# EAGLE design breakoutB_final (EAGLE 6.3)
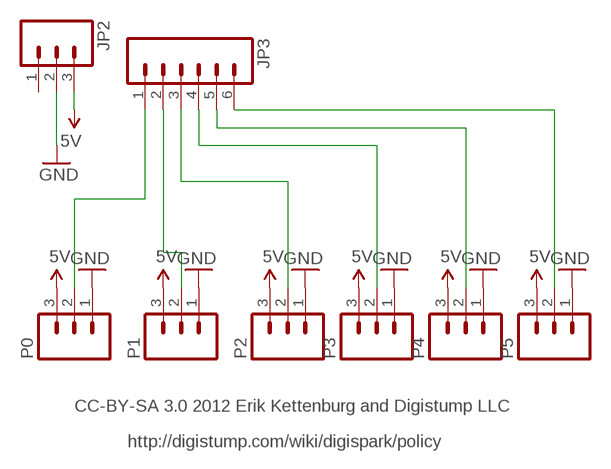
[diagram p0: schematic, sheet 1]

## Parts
JP2  M03PTH  [1X03]
JP3  M06SIP  [1X06]
P0  M03PTH  [1X03]
P1  M03PTH  [1X03]
P2  M03PTH  [1X03]
P3  M03PTH  [1X03]
P4  M03PTH  [1X03]
P5  M03PTH  [1X03]

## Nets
5V: JP2.3 P0.3 P1.3 P2.3 P3.3 P4.3 P5.3
GND: JP2.2 P0.1 P1.1 P2.1 P3.1 P4.1 P5.1
N$1: JP3.1 P0.2
N$2: JP3.2 P1.2
N$3: JP3.3 P2.2
N$4: JP3.4 P3.2
N$5: JP3.5 P4.2
N$6: JP3.6 P5.2
Unconnected: JP2.1

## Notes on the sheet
- CC-BY-SA 3.0 2012 Erik Kettenburg and Digistump LLC
- http://digistump.com/wiki/digispark/policy

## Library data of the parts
JP2 P0 P1-P5 = SparkFun:M03: Header 3 Standard 3-pin 0.1" header. Use with straight break away headers (SKU : PRT-00116), right angle break away headers (PRT-00553), swiss pins (PRT-00743), machine pins (PRT-00117), and female headers (PRT-00115). Molex polarized connector foot print use with SKU : PRT-08232 with associated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
JP3 = SparkFun:M06: Header 6 Standard 6-pin 0.1" header. Use with straight break away headers (SKU : PRT-00116), right angle break away headers (PRT-00553), swiss pins (PRT-00743), machine pins (PRT-00117), and female headers (PRT-00115). Molex polarized connector foot print use with SKU : PRT-08094 with associated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

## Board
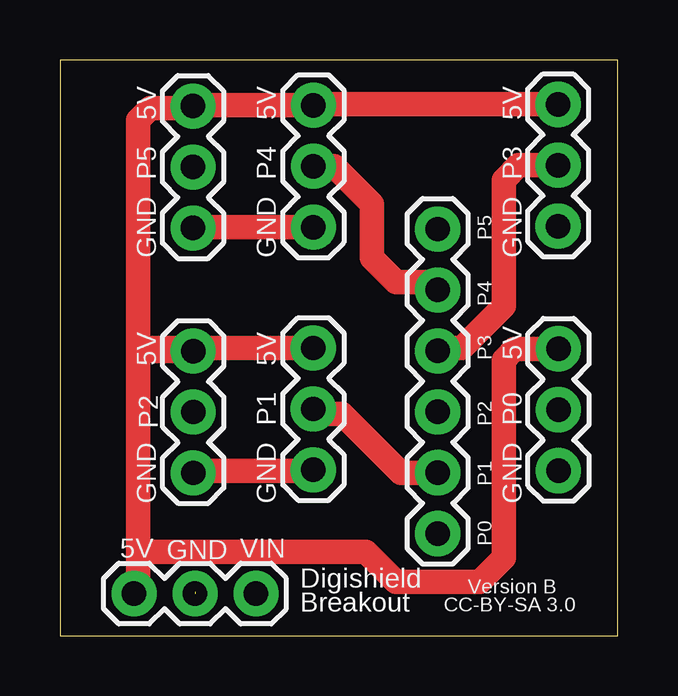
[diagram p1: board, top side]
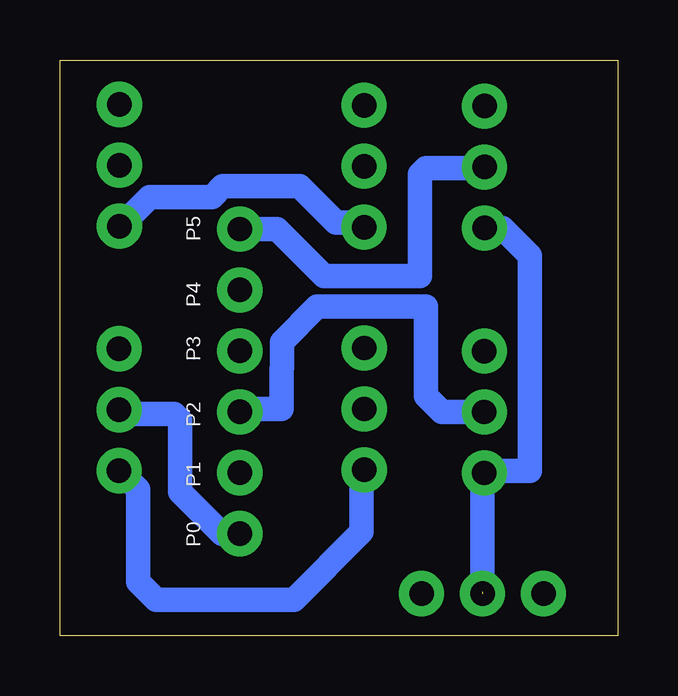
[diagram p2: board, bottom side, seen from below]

Size 23.25 x 24 mm. Coordinates in mm from the lower left corner, seen from the top.
Outline: 0,24 0,0 23.25,0 23.25,24 0,24
Copper layers (1*16): Top 0.0356mm / dielectric 1.5011mm / Bottom 0.0356mm
Design rules "default": minimum track width 40mil, minimum drill 40mil, track to track 8mil, track to pad 8mil, pad to pad 8mil, via to via 8mil, smd to smd 8mil, copper to edge 15mil, drill to drill 12mil, minimum pad ring 7mil, minimum via ring 7mil, stop-mask expansion 4mil, vias tented up to drill 25mil, thermal gap 10mil

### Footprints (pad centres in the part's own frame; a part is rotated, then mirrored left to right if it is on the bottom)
1X03 = drill 1.016 pad 1.88: 1 0,0; 2 2.54,0; 3 5.08,0
1X06 = drill 1.016 pad 1.88: 1 0,0; 2 2.54,0; 3 5.08,0; 4 7.62,0; 5 10.16,0; 6 12.7,0

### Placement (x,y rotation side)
JP2  8.17,1.75 180 top
JP3  15.75,4.25 90 top
P0  20.79,6.88 90 top
P1  10.56,6.91 90 top
P2  5.56,6.78 90 top
P3  20.77,17.07 90 top
P4  10.57,17.03 90 top
P5  5.55,17 90 top

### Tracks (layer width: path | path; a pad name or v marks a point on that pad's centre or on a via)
5V
  Top 1.016: P3.3 10.57,22.15 P4.3 5.55,22.11 P5.3 5.47,22 3.75,22 3.25,21.5 3.25,11.75 | 3.36,11.86 P2.3 5.56,11.99 P1.3 3.49,11.99 3.36,11.86 | 3.36,11.86 3.25,11.75 | 3.25,11.75 3.25,3.25 | 3.25,3.25 3.25,1.91 JP2.3 | P0.3 18.96,11.96 18.5,11.5 18.5,3.25 17.5,2.25 14,2.25 12.75,3.5 3.5,3.5 3.25,3.25
GND  (1 unrouted)
  Top 1.016: P1.1 10.52,6.86 5.64,6.86 P2.1 5.64,6.4 | P4.1 5.58,17.03 P5.1
  Bottom 1.016: 5.64,17.07 P5.1 4.8,17 3.66,15.85 3.66,6.86 5.49,6.86 P2.1 5.64,6.7 5.64,1.83 | 10.52,17.07 P4.1 10.97,17.22 11.73,17.22 13.26,18.75 16.46,18.75 16.92,18.29 19.51,18.29 20.73,17.07 P3.1 | P0.1 20,6.09 20,2.25 19.25,1.5 13.5,1.5 10.67,4.33 10.67,6.8 P1.1
N$1
  Bottom 1.016: JP3.1 16.5,4.25 18.25,6 18.25,9 18.5,9.25 20.62,9.25 P0.2
N$2
  Top 1.016: JP3.2 14.21,6.79 11.75,9.25 10.76,9.25 P1.2
N$3
  Bottom 1.016: JP3.3 15.7,9.45 14.02,9.45 14.02,11.12 14,11.15 14,12.25 12.53,13.72 8,13.72 8,10 7.32,9.32 P2.2
N$4
  Top 1.016: P3.2 19.11,19.61 18.5,19 18.5,13.75 16.75,12 15.88,12 JP3.4
N$5
  Top 1.016: P4.2 11.43,19.57 13,18 13,15.75 14,14.75 15.41,14.75 JP3.5
N$6
  Bottom 1.016: JP3.6 14.2,16.95 12.25,15 8.25,15 8.25,19.25 8,19.5 5.58,19.5 P5.2

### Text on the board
tPlace: Digishield | Version B | CC-BY-SA 3.0
tNames: 5V | 5V | 5V | P5 | P4 | P3 | GND | GND | P5 | GND | P4 | P3 | 5V | 5V | 5V | P2 | P1 | P2 | P0 | GND | GND | P1 | GND | GND | P0 | 5V | VIN | Breakout
bNames: P5 | P4 | P3 | P2 | P1 | P0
